(* Logix 5000 Rung export; software revision 16.03 *)

MODULES
   Local : vendor None type None code None
   DPS : vendor None type None code None
END_MODULES

TYPE DPS_MODULE_DEF :
STRUCT
   AppConstPattern : APP_CONSTANT_PATTERN;   // Constant Values used for DPV1 Alarm and ExtDiagData
   AppCtrl : APP_DPV1_PROG_CONTROL;   // Program Control Bits
   AppStatCnt : APP_DPV1_STAT_COUNTER;   // DPV1 Status Counter
   DiagCnf : DPS_DIAGNOSTIC_CONFIRM;   // DPS Diagnostics Confirmation
   DiagReq : DPS_DIAGNOSTIC_REQUEST;   // DPS Diagnostics Request
   DpsInputArray : DPS_INPUT_ARRAY;   // DPS Input Array
   DpsOutputArray : DPS_OUTPUT_ARRAY;   // DPS Output Array
   Dpv1AlarmCnf : DPS_DPV1C1_ALARM_CONFIRM;   // DPV1 Alarm Confirmation
   Dpv1AlarmReq : DPS_DPV1C1_ALARM_REQUEST;   // DPV1 Alarm Request
   DPV1RWDataBuffer : SINT[240];   // Buffer for DPV1 Data
   Dpv1RWRespCnf : DPS_DPV1C1_RW_RESP_CONFIRM;   // DPV1 Class 1 Read/Write Confirmation
   Dpv1RWRespReq : DPS_DPV1C1_RW_RESP_REQUEST;   // DPV1 Class 1 Read/Write Response Request
END_STRUCT
END_TYPE

TYPE DPS_DPV1C1_RW_RESP_CONFIRM :   // DPV1 Class 1 Read/Write Confirmation
STRUCT
   Reserved1 : INT;   // Reserved
   Reserved2 : INT;   // Reserved
   Answer : SINT;   // DPV1 R/W Answer
   Failure : SINT;   // DPV1 R/W Failure
   Reserved3 : INT;   // Reserved
   RwResp : SINT;   // Read Resp (=1) or Write Resp (=2)
   Reserved4 : SINT;   // Reserved
   MaAdr : SINT;   // Reply of reqesting Master Address
   Slot : SINT;   // Reply of requested Slot Number
   Index : SINT;   // Reply of requested Index
   DataLen : SINT;   // Number of requested data
   ErrCode1 : SINT;   // Reply of Error code 1 according to DPV1
   ErrCode2 : SINT;   // Reply of Error code 2 according to DPV1
   RWRespData : SINT[240];   // DPV1 Write data
END_STRUCT
END_TYPE

TYPE APP_CONSTANT_PATTERN :   // Constant Values Used for DPV1 Alarm and ExtDiagData
STRUCT
   UserAlarmData : SINT[32];   // Constants for Alarm Data
END_STRUCT
END_TYPE

TYPE DPS_DPV1C1_ALARM_CONFIRM :   // DPV1 Alarm Confirmation
STRUCT
   Reserved1 : INT;   // Reserved
   Reserved2 : INT;   // Reserved
   Answer : SINT;   // DPV1 Alarm Answer Flag
   Failure : SINT;   // DPV1 Alarm Failure
   Reserved3 : INT;   // Reserved
   Reserved4 : INT;   // Reserved
   SlotNumber : INT;   // DPV1 Alarm Slot Number
   SequenceNumber : SINT;   // DPV1 Alarm Sequence Number
   DataCnt : SINT;   // DPV1 Alarm Data Count
   AlarmType : SINT;   // DPV1 Alarm Type
   Specifier : SINT;   // DPV1 Alarm Specifier
END_STRUCT
END_TYPE

TYPE DPS_STATUS_FIELD :   // DPS Status Field
STRUCT
   ExtStaSelect : INT;   // Extended Status Select
   ExtStaLen : INT;   // Extended Status Length
   Baudrate : INT;   // Slave Baudrate
   Busaddress : SINT;   // Slave Bus Address
   UserFlags : SINT;   // User Flags
   Ident : INT;   // Slave Ident Number
   TaskState : INT;   // Slave Task State
   InputDataLen : INT;   // Slave Input Data Length
   OutputDataLen : INT;   // Slave Output Data Length
   ErrorCount : INT;   // Slave Error Count
   LastError : SINT;   // Slave Last Error
   Pad : SINT;   // Reserved
   WatchdogTime : INT;   // Slave Watchdog Time
   IrqCounter : INT;   // Slave Interrupt Counter
   C1Ind : DPS_DPV1C1_RW_INDICATION;   // DPV1 Class 1 Indication Registers
   ExtStatusInfo : SINT[96];   // Extened Status Information
END_STRUCT
END_TYPE

TYPE DPS_DIAGNOSTIC_CONFIRM :   // DPS Diagnostics Confirmation
STRUCT
   Reserved1 : INT;   // Reserved
   Reserved2 : INT;   // Reserved
   Answer : SINT;   // Answer of Diag Req
   Failure : SINT;   // Failure
   Reserved4 : INT;   // Reserved
   Reserved5 : INT;   // Reserved
   Reserved6 : INT;   // Reserved
   Reserved7 : SINT;   // Reserved
   ExtDiagDataCnt : SINT;   // Extended Diagnostics Data Count
   Mode : SINT;   // Mode
   Function : SINT;   // Function
END_STRUCT
END_TYPE

TYPE DPS_DPV1C1_ALARM_REQUEST :   // DPV1 Alarm Request
STRUCT
   Reserved1 : INT;   // Reserved
   Reserved2 : INT;   // Reserved
   Reserved3 : INT;   // Reserved
   Command : SINT;   // DPV1 Alarm Command
   Reserved4 : SINT;   // Reserved
   Reserved5 : INT;   // Reserved
   SlotNumber : INT;   // DPV1 Alarm Slot Number
   SequenceNumber : SINT;   // DPV1 Alarm Sequence Number
   DataCnt : SINT;   // DPV1 Alarm Data Count
   AlarmType : SINT;   // DPV1 Alarm Type
   Specifier : SINT;   // DPV1 Alarm Specifier
   AlarmData : SINT[28];   // DPV1 Alarm Data Array
END_STRUCT
END_TYPE

TYPE DPS_OUTPUT_ARRAY :   // DPS Output Array
STRUCT
   DevCmdReg : DPS_DEV_COMMAND_REGISTER;   // Device Command Register
   PBInputData : SINT[244];   // PROFIBIBUS Input Data for Master
END_STRUCT
END_TYPE

TYPE APP_DPV1_STAT_COUNTER :   // DPV1 Status Counter
STRUCT
   NumReadWrite : DINT;   // Number of DPV1 Read Write Response Sent
   ReadRespPos : DINT;   // Number of DPV1 Read Response Successful
   ReadRespNeg : DINT;   // Number of DPV1 Read Response Failed
   WriteRespPos : DINT;   // Number of DPV1 Write Response Successful
   WriteRespNeg : DINT;   // Number of DPV1 Write Response Failed
   NumAlarmRequest : DINT;   // Number of DPV1 Alarm Requests sent
   AlarmRequestPos : DINT;   // Number of DPV1 Alarm Requests Successful
   AlarmRequestNeg : DINT;   // Number of DPV1 Alarm Requests Failed
   NumDiagReq : DINT;   // Number of Diagnostic Reports Sent
   DiagReqPos : DINT;   // Number of Diagnostic Report Successful
   DiagReqNeg : DINT;   // Number of Diagnostic Report Failed
END_STRUCT
END_TYPE

TYPE DPS_DEV_COMMAND_REGISTER :   // Device Command Register
STRUCT
   Reserved0 : BOOL;   // Reserved
   Reserved1 : BOOL;   // Reserved
   Reserved2 : BOOL;   // Reserved
   Reserved3 : BOOL;   // Reserved
   Reserved4 : BOOL;   // Reserved
   NRdy : BOOL;   // Application Not Ready
   Init : BOOL;   // Init ( Warm boot )
   Reset : BOOL;   // Reset ( Cold boot )
   Reserved5 : SINT;   // Reserved
   Reserved6 : SINT;   // Reserved
   ExtStaSelect : SINT;   // Extra Status Select
END_STRUCT
END_TYPE

TYPE DPS_FW_REVISION :   // Firmware Major/Minor Revision
STRUCT
   FwMinor : SINT;   // Firmware Minor Revison
   FwMajor : SINT;   // Firmware Major Revison
   Reserved : INT;   // Reserved
END_STRUCT
END_TYPE

TYPE APP_DPV1_PROG_CONTROL :   // Program Control Bits
STRUCT
   MainInitDone : BOOL;   // Main Initialization Complete
   Dpv1ReadRespInProgress : BOOL;   // DPV1 Read Response in Progress
   Dpv1WriteRespInProgress : BOOL;   // DPV1 Write Response in Progress
   Dpv1AlarmReqSend : BOOL;   // DPV1 Alarm Request Flag
   Dpv1AlarmReqInProgress : BOOL;   // DPV1 Alarm Request in Progress
   DpsDiagReqSend : BOOL;   // DPS Diagnostics Request Flag
   DpsDiagReqInProgress : BOOL;   // DPS Diagnostic Request in Progress
   Reserved0 : BOOL;   // Reserved
   Reserved1 : BOOL;   // Reserved
   Reserved2 : BOOL;   // Reserved
   Reserved3 : BOOL;   // Reserved
   Reserved4 : BOOL;   // Reserved
   Reserved5 : BOOL;   // Reserved
   Reserved6 : BOOL;   // Reserved
   Reserved7 : BOOL;   // Reserved
   Reserved8 : BOOL;   // Reserved
   DPV1RWIndCnt : SINT;   // DPV1 R/W Indication Counter
END_STRUCT
END_TYPE

TYPE DPS_DPV1C1_RW_RESP_REQUEST :   // DPV1 Class 1 Read/Write Response Request
STRUCT
   Reserved1 : INT;   // Reserved
   Reserved2 : INT;   // Reserved
   Reserved3 : INT;   // Reserved
   Command : SINT;   // DPV1 ReadWrite Resp. Request (=17)
   Reserved4 : SINT;   // Reserved
   RwResp : SINT;   // Read Resp (=1) or Write Resp (=2)
   Reserved5 : SINT;   // Reserved
   MaAdr : SINT;   // Reply of reqesting Master Address
   Slot : SINT;   // Reply of requested Slot Number
   Index : SINT;   // Reply of requested Index
   DataLen : SINT;   // Reply of requested number of data
   ErrCode1 : SINT;   // Error code 1 according to DPV1
   ErrCode2 : SINT;   // Error code 2 according to DPV1
   RWRespData : SINT[240];   // DPV1 Read response data
END_STRUCT
END_TYPE

TYPE DPS_DIAGNOSTIC_REQUEST :   // DPS Diagnostics Request
STRUCT
   Reserved1 : INT;   // Reserved
   Reserved2 : INT;   // Reserved
   Reserved3 : INT;   // Reserved
   Command : SINT;   // Command for Diag Req = 24
   Reserved4 : SINT;   // Reserved
   Reserved5 : INT;   // Reserved
   Reserved6 : INT;   // Reserved
   Reserved7 : SINT;   // Reserved
   ExtDiagDataCnt : SINT;   // Number of ext. diag data
   Mode : SINT;   // Diag mode: (0 = default, 1 = suppress Ext.DiagBit)
   Function : SINT;   // Send diag once (fix 18)
   DiagData : SINT[32];   // Extended diag data (format see PROFIBUS Norm)
END_STRUCT
END_TYPE

TYPE DPS_DPV1C1_RW_INDICATION :   // DPV1 C1 Read/Write Indication
STRUCT
   ReadReq : BOOL;   // Indicates a Read request
   WriteReq : BOOL;   // Indicates a Write request
   Reserved2 : BOOL;   // Reserved
   Reserved3 : BOOL;   // Reserved
   Reserved4 : BOOL;   // Reserved
   Reserved5 : BOOL;   // Reserved
   Reserved6 : BOOL;   // Reserved
   Reserved7 : BOOL;   // Reserved
   RwCnt : SINT;   // ReadWrite indication counter
   MaAdr : SINT;   // Address of reqesting master
   Slot : SINT;   // Requested Slot Number
   Index : SINT;   // Requested Index
   DataLen : SINT;   // Requested Data Length
   Reserved8 : SINT;   // Reserved
   Reserved9 : SINT;   // Reserved
END_STRUCT
END_TYPE

TYPE DPS_INPUT_ARRAY :   // DPS Input Array
STRUCT
   DevStaReg : DPS_DEV_STATUS_REGISTER;   // Device Status Registers
   FwRev : DPS_FW_REVISION;   // Firmware Revision
   StaField : DPS_STATUS_FIELD;   // DPS Status Registers
   PBOutputData : SINT[380];   // PROFIBUS Output Data from Matser
END_STRUCT
END_TYPE

TYPE DPS_DEV_STATUS_REGISTER :   // Device Status Register
STRUCT
   Reserved0 : BOOL;   // Reserved
   Reserved1 : BOOL;   // Reserved
   Reserved2 : BOOL;   // Reserved
   Reserved3 : BOOL;   // Reserved
   Reserved4 : BOOL;   // Reserved
   Com : BOOL;   // Communication
   Run : BOOL;   // Running
   Rdy : BOOL;   // Ready
   Reserved5 : SINT;   // Reserved
   Reserved6 : SINT;   // Reserved
   Reserved7 : SINT;   // Reserved
END_STRUCT
END_TYPE

ADD_ON_INSTRUCTION AOIPS69DPS   (* revision 1.1, vendor Prosoft Technology Inc *)
// Add-On instruction for the PS69-DPS module
// Revision note:
// Added viewing capability for the Add_On Instruction
VAR_IN_OUT
   Connection_Input : INT[190]; {required}   // Connect to module input image
   Connection_Output : INT[124]; {required}   // Connect to module output image
   PS69DPS : DPS_MODULE_DEF; {required}   // Main controller tag
   DiagReqMsg : MESSAGE; {required}
   Dpv1AlarmMsg : MESSAGE; {required}
   Dpv1RWMsg : MESSAGE; {required}
END_VAR

ROUTINE Logic   (* ladder *)
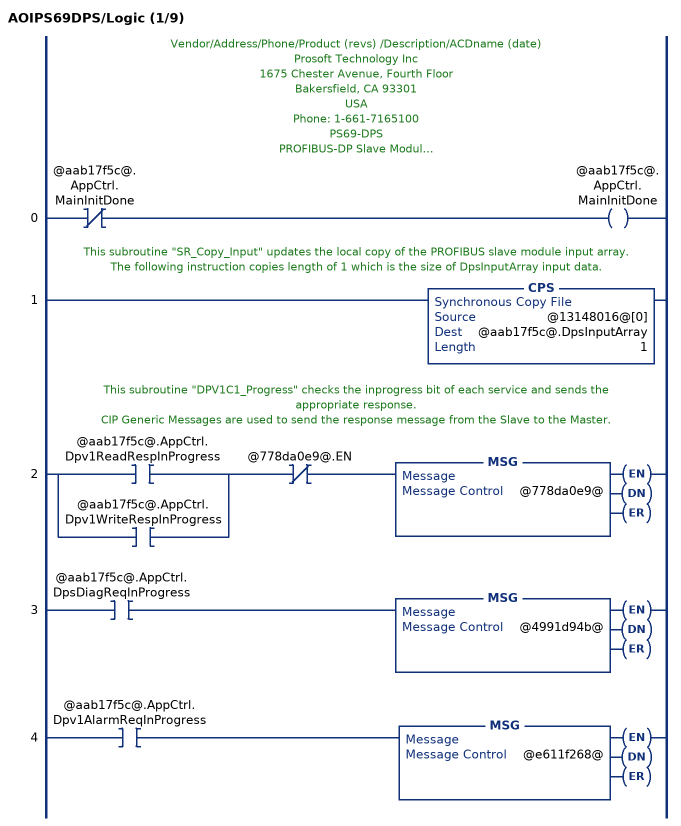
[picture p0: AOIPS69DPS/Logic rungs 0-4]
   // Vendor/Address/Phone/Product (revs) /Description/ACDname (date)
   // Prosoft Technology Inc
   // 1675 Chester Avenue, Fourth Floor
   // Bakersfield, CA 93301
   // USA
   // Phone: 1-661-7165100
   // PS69-DPS
   // PROFIBUS-DP Slave Module
   // PS69_DPS_messaging_L32E.ACD (Rev1.0) (07/28/05)
   // Although this program has been developed with great care and intensively tested,
   // Prosoft Technology Inc cannot guarantee the suitability of this program
   // for any purpose not confirmed by us in writing.
   // We reserve the right to modify our products and their specifications at any time in as far as this contributes to technical progress.
   // The version of the manual supplied with the program applies.
   // This program is a basic example RSLogix5000 project used for sending PROFIBUS messages to the communication module "PS69-DPS". This project provides an example for every supported PROFIBUS message by the module.
   // For detailed information about the these messages (functionality, parameters, error codes etc. ) refer to the module User Manual document.
   // This Rung calls all init routines for one time, to initialize the PROFIBUS commands.
   0: XIO(@aab17f5c@.AppCtrl.MainInitDone)OTE(@aab17f5c@.AppCtrl.MainInitDone);
   // This subroutine "SR_Copy_Input" updates the local copy of the PROFIBUS slave module input array.
   // The following instruction copies length of 1 which is the size of DpsInputArray input data.
   1: CPS(@13148016@[0],@aab17f5c@.DpsInputArray,1);
   // This subroutine "DPV1C1_Progress" checks the inprogress bit of each service and sends the appropriate response.
   // CIP Generic Messages are used to send the response message from the Slave to the Master.
   2: [XIC(@aab17f5c@.AppCtrl.Dpv1ReadRespInProgress) ,XIC(@aab17f5c@.AppCtrl.Dpv1WriteRespInProgress) ]XIO(@778da0e9@.EN)MSG(@778da0e9@);
   3: XIC(@aab17f5c@.AppCtrl.DpsDiagReqInProgress)MSG(@4991d94b@);
   4: XIC(@aab17f5c@.AppCtrl.Dpv1AlarmReqInProgress)MSG(@e611f268@);
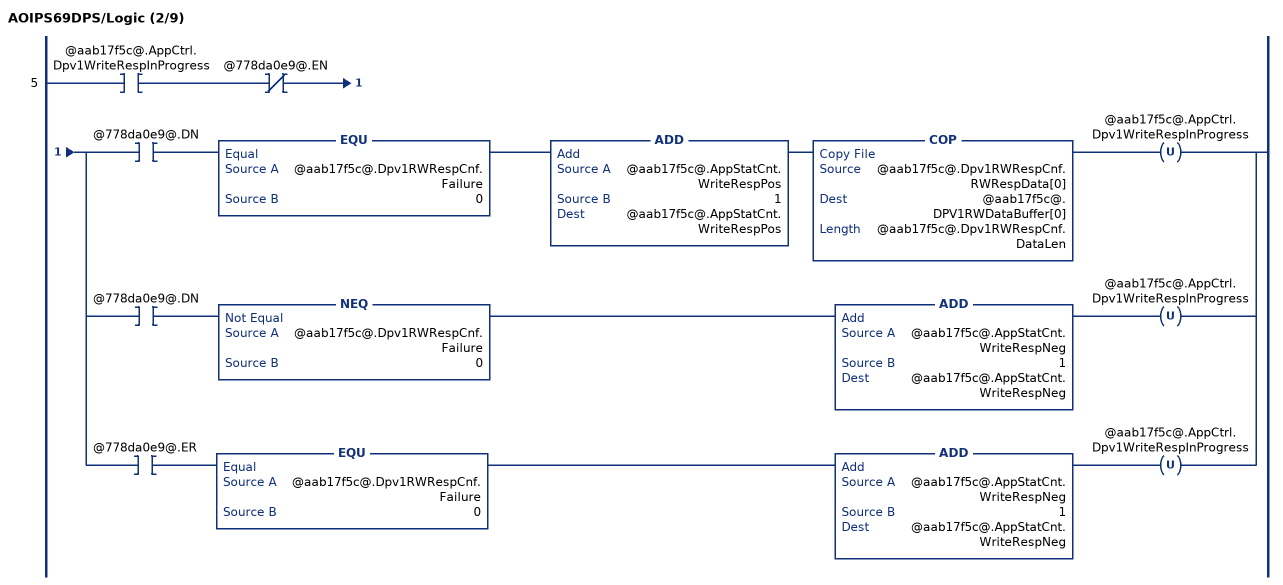
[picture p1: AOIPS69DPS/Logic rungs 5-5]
   5: XIC(@aab17f5c@.AppCtrl.Dpv1WriteRespInProgress)XIO(@778da0e9@.EN)[XIC(@778da0e9@.DN) EQU(@aab17f5c@.Dpv1RWRespCnf.Failure,0) ADD(@aab17f5c@.AppStatCnt.WriteRespPos,1,@aab17f5c@.AppStatCnt.WriteRespPos) COP(@aab17f5c@.Dpv1RWRespCnf.RWRespData[0],@aab17f5c@.DPV1RWDataBuffer[0],@aab17f5c@.Dpv1RWRespCnf.DataLen) OTU(@aab17f5c@.AppCtrl.Dpv1WriteRespInProgress) ,XIC(@778da0e9@.DN) NEQ(@aab17f5c@.Dpv1RWRespCnf.Failure,0) ADD(@aab17f5c@.AppStatCnt.WriteRespNeg,1,@aab17f5c@.AppStatCnt.WriteRespNeg) OTU(@aab17f5c@.AppCtrl.Dpv1WriteRespInProgress) ,XIC(@778da0e9@.ER) EQU(@aab17f5c@.Dpv1RWRespCnf.Failure,0) ADD(@aab17f5c@.AppStatCnt.WriteRespNeg,1,@aab17f5c@.AppStatCnt.WriteRespNeg) OTU(@aab17f5c@.AppCtrl.Dpv1WriteRespInProgress) ];
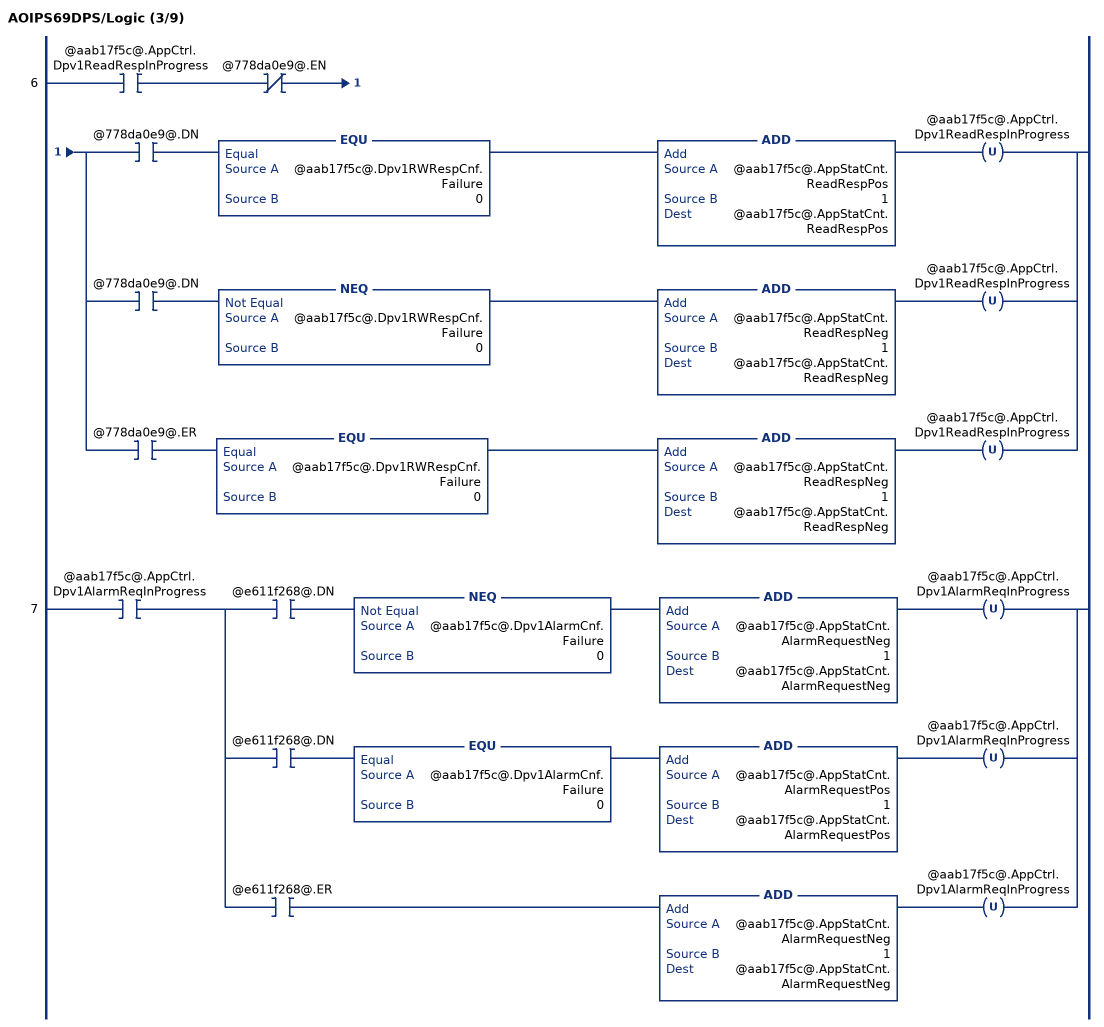
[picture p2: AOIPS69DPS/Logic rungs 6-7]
   6: XIC(@aab17f5c@.AppCtrl.Dpv1ReadRespInProgress)XIO(@778da0e9@.EN)[XIC(@778da0e9@.DN) EQU(@aab17f5c@.Dpv1RWRespCnf.Failure,0) ADD(@aab17f5c@.AppStatCnt.ReadRespPos,1,@aab17f5c@.AppStatCnt.ReadRespPos) OTU(@aab17f5c@.AppCtrl.Dpv1ReadRespInProgress) ,XIC(@778da0e9@.DN) NEQ(@aab17f5c@.Dpv1RWRespCnf.Failure,0) ADD(@aab17f5c@.AppStatCnt.ReadRespNeg,1,@aab17f5c@.AppStatCnt.ReadRespNeg) OTU(@aab17f5c@.AppCtrl.Dpv1ReadRespInProgress) ,XIC(@778da0e9@.ER) EQU(@aab17f5c@.Dpv1RWRespCnf.Failure,0) ADD(@aab17f5c@.AppStatCnt.ReadRespNeg,1,@aab17f5c@.AppStatCnt.ReadRespNeg) OTU(@aab17f5c@.AppCtrl.Dpv1ReadRespInProgress) ];
   7: XIC(@aab17f5c@.AppCtrl.Dpv1AlarmReqInProgress)[XIC(@e611f268@.DN) NEQ(@aab17f5c@.Dpv1AlarmCnf.Failure,0) ADD(@aab17f5c@.AppStatCnt.AlarmRequestNeg,1,@aab17f5c@.AppStatCnt.AlarmRequestNeg) OTU(@aab17f5c@.AppCtrl.Dpv1AlarmReqInProgress) ,XIC(@e611f268@.DN) EQU(@aab17f5c@.Dpv1AlarmCnf.Failure,0) ADD(@aab17f5c@.AppStatCnt.AlarmRequestPos,1,@aab17f5c@.AppStatCnt.AlarmRequestPos) OTU(@aab17f5c@.AppCtrl.Dpv1AlarmReqInProgress) ,XIC(@e611f268@.ER) ADD(@aab17f5c@.AppStatCnt.AlarmRequestNeg,1,@aab17f5c@.AppStatCnt.AlarmRequestNeg) OTU(@aab17f5c@.AppCtrl.Dpv1AlarmReqInProgress) ];
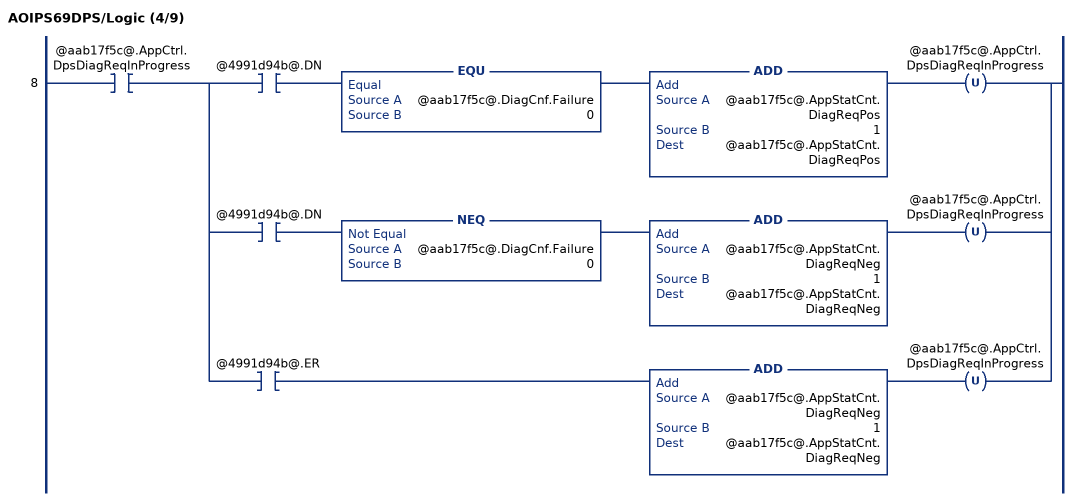
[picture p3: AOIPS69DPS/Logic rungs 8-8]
   8: XIC(@aab17f5c@.AppCtrl.DpsDiagReqInProgress)[XIC(@4991d94b@.DN) EQU(@aab17f5c@.DiagCnf.Failure,0) ADD(@aab17f5c@.AppStatCnt.DiagReqPos,1,@aab17f5c@.AppStatCnt.DiagReqPos) OTU(@aab17f5c@.AppCtrl.DpsDiagReqInProgress) ,XIC(@4991d94b@.DN) NEQ(@aab17f5c@.DiagCnf.Failure,0) ADD(@aab17f5c@.AppStatCnt.DiagReqNeg,1,@aab17f5c@.AppStatCnt.DiagReqNeg) OTU(@aab17f5c@.AppCtrl.DpsDiagReqInProgress) ,XIC(@4991d94b@.ER) ADD(@aab17f5c@.AppStatCnt.DiagReqNeg,1,@aab17f5c@.AppStatCnt.DiagReqNeg) OTU(@aab17f5c@.AppCtrl.DpsDiagReqInProgress) ];
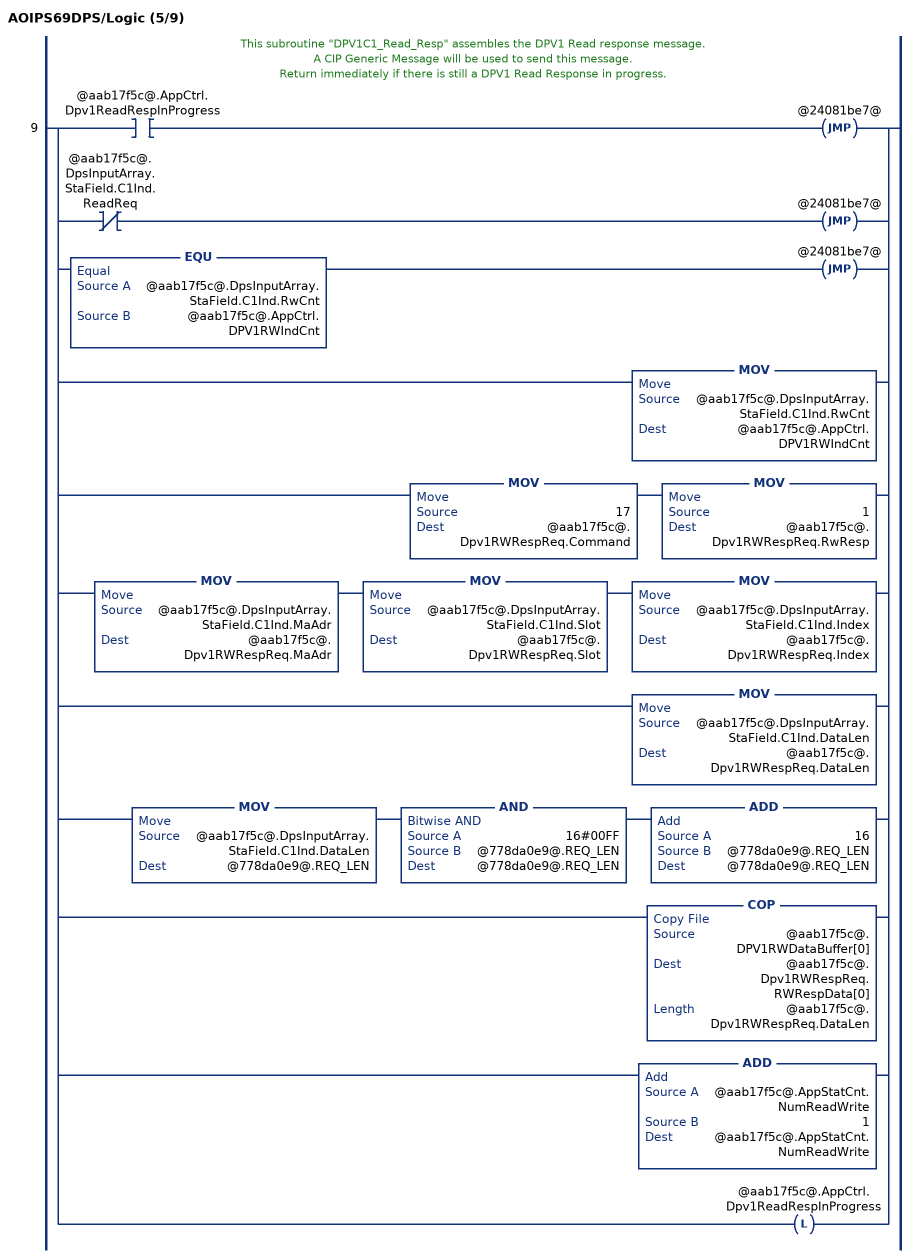
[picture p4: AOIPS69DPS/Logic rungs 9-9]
   // This subroutine "DPV1C1_Read_Resp" assembles the DPV1 Read response message.
   // A CIP Generic Message will be used to send this message.
   // Return immediately if there is still a DPV1 Read Response in progress.
   9: [XIC(@aab17f5c@.AppCtrl.Dpv1ReadRespInProgress) JMP(@24081be7@) ,XIO(@aab17f5c@.DpsInputArray.StaField.C1Ind.ReadReq) JMP(@24081be7@) ,EQU(@aab17f5c@.DpsInputArray.StaField.C1Ind.RwCnt,@aab17f5c@.AppCtrl.DPV1RWIndCnt) JMP(@24081be7@) ,MOV(@aab17f5c@.DpsInputArray.StaField.C1Ind.RwCnt,@aab17f5c@.AppCtrl.DPV1RWIndCnt) ,MOV(17,@aab17f5c@.Dpv1RWRespReq.Command) MOV(1,@aab17f5c@.Dpv1RWRespReq.RwResp) ,MOV(@aab17f5c@.DpsInputArray.StaField.C1Ind.MaAdr,@aab17f5c@.Dpv1RWRespReq.MaAdr) MOV(@aab17f5c@.DpsInputArray.StaField.C1Ind.Slot,@aab17f5c@.Dpv1RWRespReq.Slot) MOV(@aab17f5c@.DpsInputArray.StaField.C1Ind.Index,@aab17f5c@.Dpv1RWRespReq.Index) ,MOV(@aab17f5c@.DpsInputArray.StaField.C1Ind.DataLen,@aab17f5c@.Dpv1RWRespReq.DataLen) ,MOV(@aab17f5c@.DpsInputArray.StaField.C1Ind.DataLen,@778da0e9@.REQ_LEN) AND(16#00FF,@778da0e9@.REQ_LEN,@778da0e9@.REQ_LEN) ADD(16,@778da0e9@.REQ_LEN,@778da0e9@.REQ_LEN) ,COP(@aab17f5c@.DPV1RWDataBuffer[0],@aab17f5c@.Dpv1RWRespReq.RWRespData[0],@aab17f5c@.Dpv1RWRespReq.DataLen) ,ADD(@aab17f5c@.AppStatCnt.NumReadWrite,1,@aab17f5c@.AppStatCnt.NumReadWrite) ,OTL(@aab17f5c@.AppCtrl.Dpv1ReadRespInProgress) ];
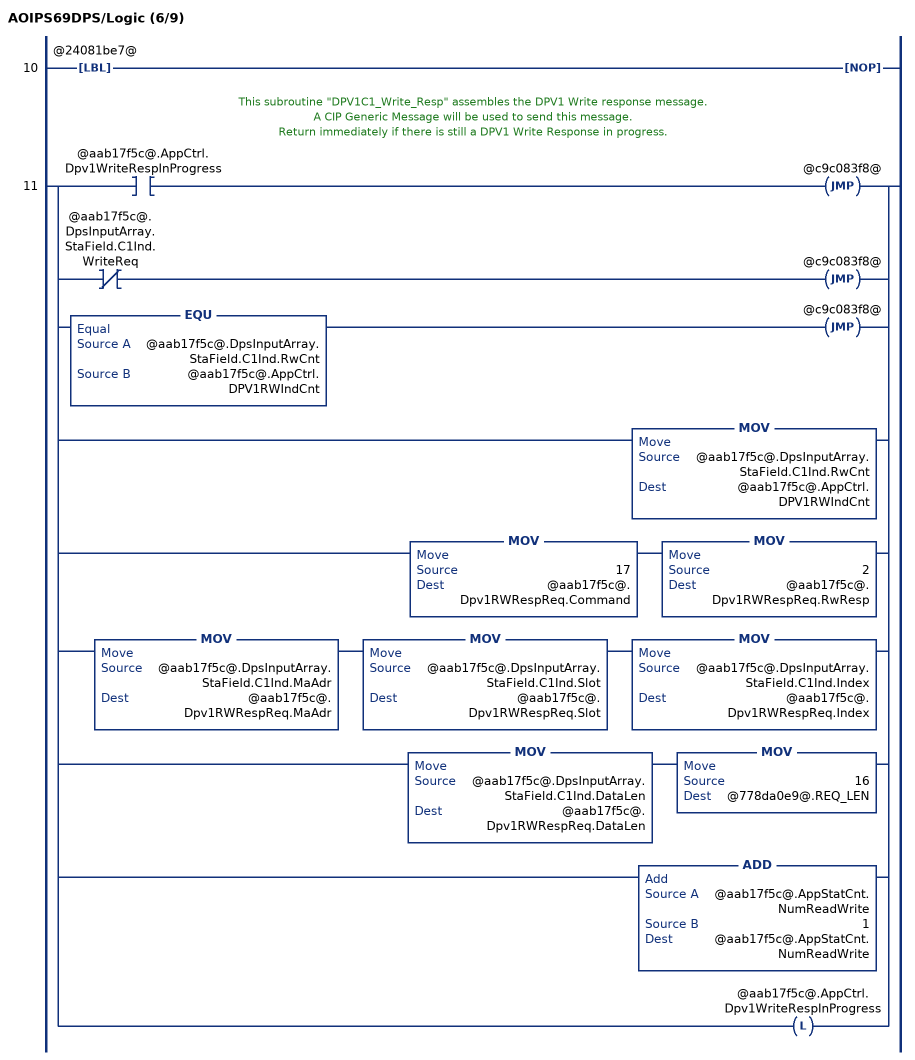
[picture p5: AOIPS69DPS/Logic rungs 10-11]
   10: LBL(@24081be7@)NOP();
   // This subroutine "DPV1C1_Write_Resp" assembles the DPV1 Write response message.
   // A CIP Generic Message will be used to send this message.
   // Return immediately if there is still a DPV1 Write Response in progress.
   11: [XIC(@aab17f5c@.AppCtrl.Dpv1WriteRespInProgress) JMP(@c9c083f8@) ,XIO(@aab17f5c@.DpsInputArray.StaField.C1Ind.WriteReq) JMP(@c9c083f8@) ,EQU(@aab17f5c@.DpsInputArray.StaField.C1Ind.RwCnt,@aab17f5c@.AppCtrl.DPV1RWIndCnt) JMP(@c9c083f8@) ,MOV(@aab17f5c@.DpsInputArray.StaField.C1Ind.RwCnt,@aab17f5c@.AppCtrl.DPV1RWIndCnt) ,MOV(17,@aab17f5c@.Dpv1RWRespReq.Command) MOV(2,@aab17f5c@.Dpv1RWRespReq.RwResp) ,MOV(@aab17f5c@.DpsInputArray.StaField.C1Ind.MaAdr,@aab17f5c@.Dpv1RWRespReq.MaAdr) MOV(@aab17f5c@.DpsInputArray.StaField.C1Ind.Slot,@aab17f5c@.Dpv1RWRespReq.Slot) MOV(@aab17f5c@.DpsInputArray.StaField.C1Ind.Index,@aab17f5c@.Dpv1RWRespReq.Index) ,MOV(@aab17f5c@.DpsInputArray.StaField.C1Ind.DataLen,@aab17f5c@.Dpv1RWRespReq.DataLen) MOV(16,@778da0e9@.REQ_LEN) ,ADD(@aab17f5c@.AppStatCnt.NumReadWrite,1,@aab17f5c@.AppStatCnt.NumReadWrite) ,OTL(@aab17f5c@.AppCtrl.Dpv1WriteRespInProgress) ];
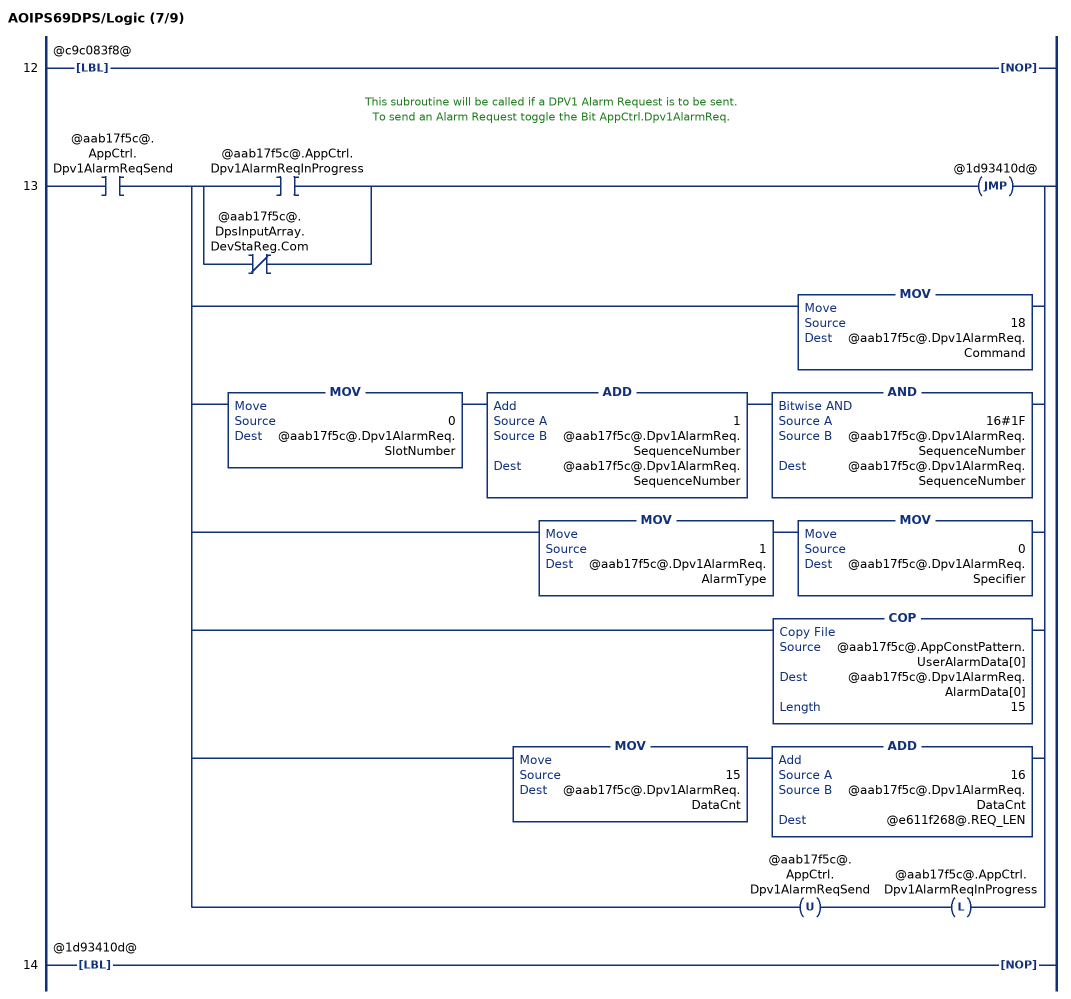
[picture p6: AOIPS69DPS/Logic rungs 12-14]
   12: LBL(@c9c083f8@)NOP();
   // This subroutine will be called if a DPV1 Alarm Request is to be sent.
   // To send an Alarm Request toggle the Bit AppCtrl.Dpv1AlarmReq.
   13: XIC(@aab17f5c@.AppCtrl.Dpv1AlarmReqSend)[[XIC(@aab17f5c@.AppCtrl.Dpv1AlarmReqInProgress) ,XIO(@aab17f5c@.DpsInputArray.DevStaReg.Com) ] JMP(@1d93410d@) ,MOV(18,@aab17f5c@.Dpv1AlarmReq.Command) ,MOV(0,@aab17f5c@.Dpv1AlarmReq.SlotNumber) ADD(1,@aab17f5c@.Dpv1AlarmReq.SequenceNumber,@aab17f5c@.Dpv1AlarmReq.SequenceNumber) AND(16#1F,@aab17f5c@.Dpv1AlarmReq.SequenceNumber,@aab17f5c@.Dpv1AlarmReq.SequenceNumber) ,MOV(1,@aab17f5c@.Dpv1AlarmReq.AlarmType) MOV(0,@aab17f5c@.Dpv1AlarmReq.Specifier) ,COP(@aab17f5c@.AppConstPattern.UserAlarmData[0],@aab17f5c@.Dpv1AlarmReq.AlarmData[0],15) ,MOV(15,@aab17f5c@.Dpv1AlarmReq.DataCnt) ADD(16,@aab17f5c@.Dpv1AlarmReq.DataCnt,@e611f268@.REQ_LEN) ,OTU(@aab17f5c@.AppCtrl.Dpv1AlarmReqSend) OTL(@aab17f5c@.AppCtrl.Dpv1AlarmReqInProgress) ];
   14: LBL(@1d93410d@)NOP();
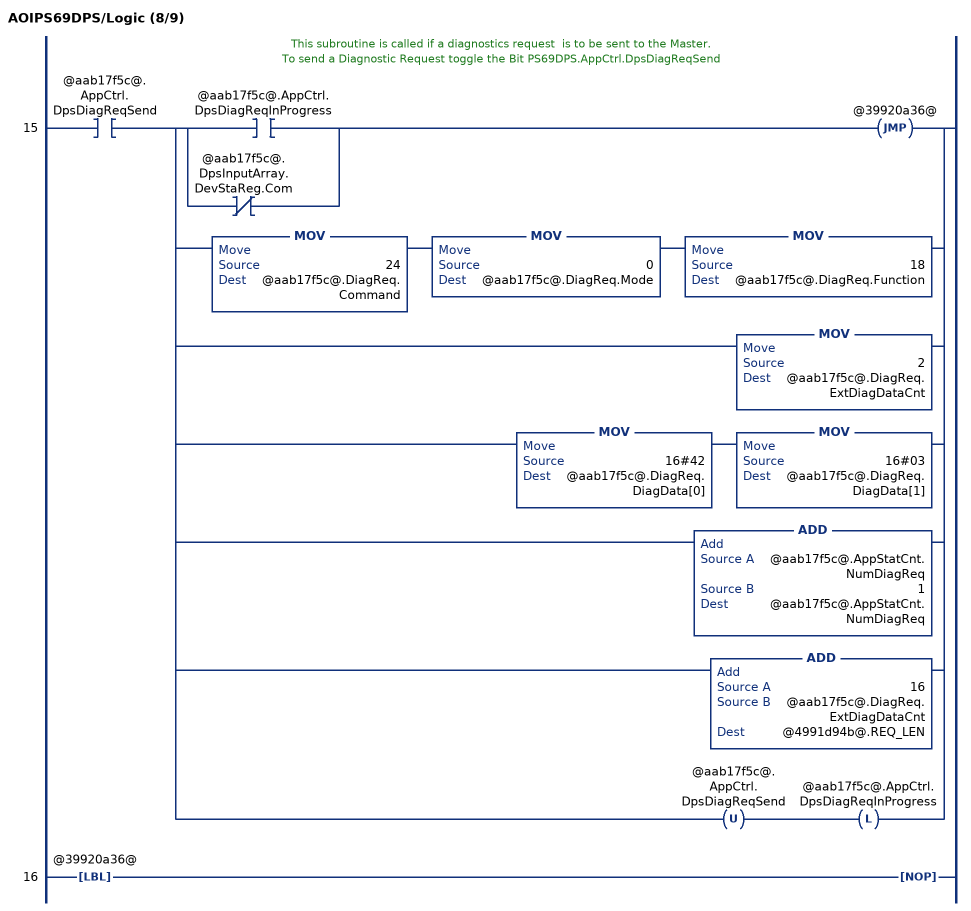
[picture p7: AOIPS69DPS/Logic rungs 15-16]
   // This subroutine is called if a diagnostics request  is to be sent to the Master.
   // To send a Diagnostic Request toggle the Bit PS69DPS.AppCtrl.DpsDiagReqSend
   15: XIC(@aab17f5c@.AppCtrl.DpsDiagReqSend)[[XIC(@aab17f5c@.AppCtrl.DpsDiagReqInProgress) ,XIO(@aab17f5c@.DpsInputArray.DevStaReg.Com) ] JMP(@39920a36@) ,MOV(24,@aab17f5c@.DiagReq.Command) MOV(0,@aab17f5c@.DiagReq.Mode) MOV(18,@aab17f5c@.DiagReq.Function) ,MOV(2,@aab17f5c@.DiagReq.ExtDiagDataCnt) ,MOV(16#42,@aab17f5c@.DiagReq.DiagData[0]) MOV(16#03,@aab17f5c@.DiagReq.DiagData[1]) ,ADD(@aab17f5c@.AppStatCnt.NumDiagReq,1,@aab17f5c@.AppStatCnt.NumDiagReq) ,ADD(16,@aab17f5c@.DiagReq.ExtDiagDataCnt,@4991d94b@.REQ_LEN) ,OTU(@aab17f5c@.AppCtrl.DpsDiagReqSend) OTL(@aab17f5c@.AppCtrl.DpsDiagReqInProgress) ];
   16: LBL(@39920a36@)NOP();
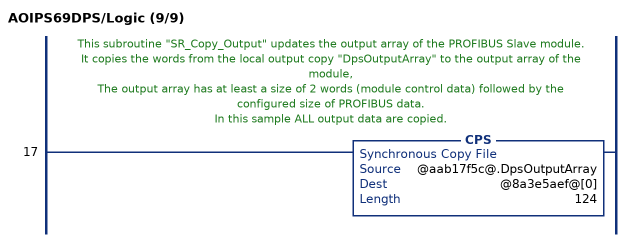
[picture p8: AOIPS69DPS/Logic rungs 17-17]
   // This subroutine "SR_Copy_Output" updates the output array of the PROFIBUS Slave module.
   // It copies the words from the local output copy "DpsOutputArray" to the output array of the module,
   // The output array has at least a size of 2 words (module control data) followed by the configured size of PROFIBUS data.
   // In this sample ALL output data are copied.
   17: CPS(@aab17f5c@.DpsOutputArray,@8a3e5aef@[0],124);
END_ROUTINE
END_ADD_ON_INSTRUCTION

VAR_GLOBAL   (* controller tags *)
   Local:1:O : AB:1769_MODULE_INT_248Bytes:O:0;
   AOIPS69DPS : AOIPS69DPS;
   PS69DPS : DPS_MODULE_DEF;
   Dpv1AlarmMsg : MESSAGE;
        MessageParameters(MessageType := CIP Generic, RequestedLength := 31, ConnectedFlag := 2, ConnectionPath := DPS, ServiceCode := 16#0064, ObjectType := 16#0065, TargetObject := 2, LocalElement := PS69DPS.Dpv1AlarmReq, DestinationTag := PS69DPS.Dpv1AlarmCnf)
   DiagReqMsg : MESSAGE;
        MessageParameters(MessageType := CIP Generic, RequestedLength := 18, ConnectedFlag := 2, ConnectionPath := DPS, ServiceCode := 16#0064, ObjectType := 16#0065, TargetObject := 2, LocalElement := PS69DPS.DiagReq, DestinationTag := PS69DPS.DiagCnf)
   Local:1:I : AB:1769_MODULE_INT_384Bytes:I:0;
   Dpv1RWMsg : MESSAGE;
        MessageParameters(MessageType := CIP Generic, RequestedLength := 1, ConnectedFlag := 2, ConnectionPath := DPS, ServiceCode := 16#0064, ObjectType := 16#0065, TargetObject := 2, LocalElement := PS69DPS.Dpv1RWRespReq, DestinationTag := PS69DPS.Dpv1RWRespCnf)
END_VAR

PROGRAM MainProgram

ROUTINE MainRoutine   (* ladder *)
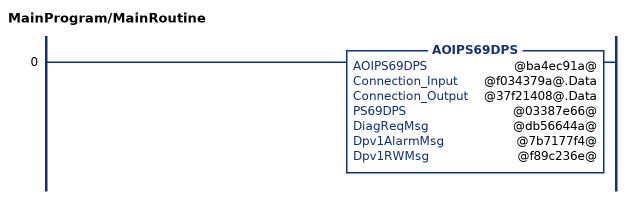
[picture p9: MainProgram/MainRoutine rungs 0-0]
   0: AOIPS69DPS(@ba4ec91a@,@f034379a@.Data,@37f21408@.Data,@03387e66@,@db56644a@,@7b7177f4@,@f89c236e@);
END_ROUTINE
END_PROGRAM
